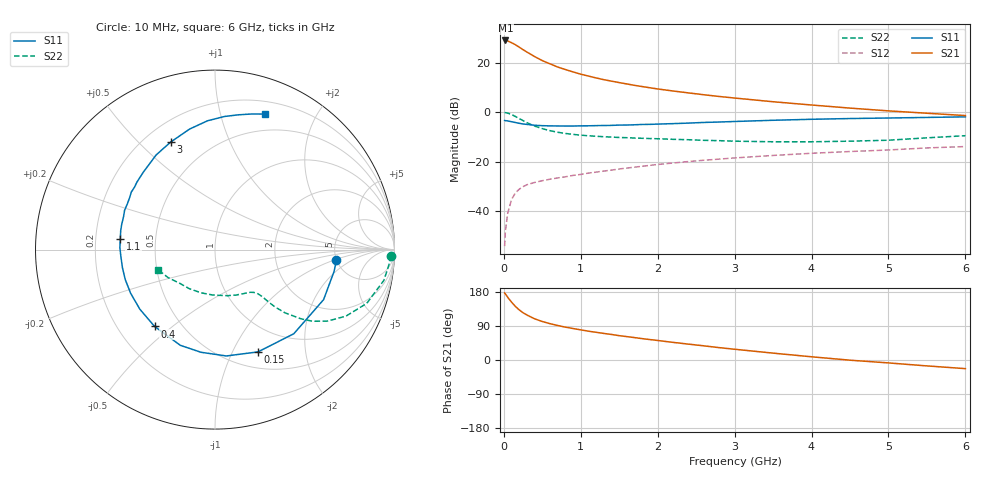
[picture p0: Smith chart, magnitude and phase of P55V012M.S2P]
! SIEMENS Small Signal Semiconductors
! BFP183
! Si NPN RF Bipolar Junction Transistor in SOT143
! VCE = 5 V  IC = 12 mA
! Common Emitter S-Parameters:  March  1996
# GHz  S  MA  R  50
!  f  S11  S21  S12  S22
! GHz  MAG  ANG  MAG  ANG  MAG  ANG  MAG  ANG
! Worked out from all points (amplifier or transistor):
!   36 points, 10 MHz to 6 GHz, reference 50 ohm
!   highest |S21| = 28.9 dB at 20 MHz (marker M1)
!   |S21| within 3 dB of that: start of sweep to 214.8 MHz
!   unconditionally stable (mu >= 1): 1.127 GHz to 5.654 GHz
!   at 250 MHz: K = 0.35, MSG = 27.6 dB, |S12| = -30.0 dB
!   at 1.4 GHz: K = 1.08, MAG = 16.2 dB, |S12| = -23.3 dB
!   at 6 GHz: K = 0.96, MSG = 6.2 dB, |S12| = -13.9 dB
!   S11 on the Smith chart (normalised r, x): 10 MHz: 5.00, -1.08; 150 MHz: 0.68, -1.26; 400 MHz: 0.36, -0.43; 1.1 GHz: 0.31, +0.05; 3 GHz: 0.30, +0.63; 6 GHz: 0.32, +1.38
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0.01  0.6794 -4.9  27.71 176.9  0.002 86.1  0.9816 -2.0
0.02  0.6746 -10.3  27.8 174.3  0.004 81.4  0.9764 -4.1
0.05  0.6662 -24.7  27.15 165.6  0.0092 80.0  0.9565 -10.3
0.1  0.6423 -46.9  25.05 152.8  0.0174 68.8  0.8971 -19.5
0.15  0.6181 -67.2  22.82 141.3  0.0236 61.4  0.8188 -26.9
0.2  0.596 -83.9  20.39 132.2  0.0281 55.7  0.7432 -32.4
0.25  0.5773 -97.8  18.11 124.7  0.0316 51.6  0.6745 -36.3
0.3  0.5672 -109.9  16.24 118.7  0.0345 48.9  0.6133 -38.9
0.4  0.5446 -128.2  13.17 108.7  0.0384 46.1  0.5251 -42.1
0.5  0.5344 -141.6  10.92 101.6  0.0417 43.8  0.4659 -43.6
0.6  0.5293 -152.6  9.399 95.9  0.0446 43.4  0.424 -44.3
0.7  0.5271 -161.4  8.113 91.0  0.0473 44.3  0.3938 -44.6
0.9  0.5254 -175.1  6.464 83.1  0.0532 44.5  0.3569 -45.3
1.1  0.5311 173.4  5.331 76.0  0.0593 45.3  0.3344 -46.5
1.5  0.5493 156.5  3.938 64.2  0.0717 45.8  0.3092 -50.2
1.8  0.5658 145.5  3.275 56.4  0.0813 45.6  0.2974 -54.6
2.2  0.5876 132.9  2.669 46.5  0.0946 44.0  0.2838 -61.6
3  0.6488 112.1  1.925 28.4  0.1198 39.1  0.2602 -79.5
3.5  0.6863 101.9  1.621 18.1  0.1343 35.6  0.2534 -92.9
4.5  0.7437 85.9  1.207 -0.5  0.1612 27.6  0.2604 -123.3
5.5  0.783 74.8  0.951 -15.6  0.1904 20.7  0.304 -149.0
6  0.8041 69.9  0.854 -22.8  0.2029 16.4  0.3357 -160.4
